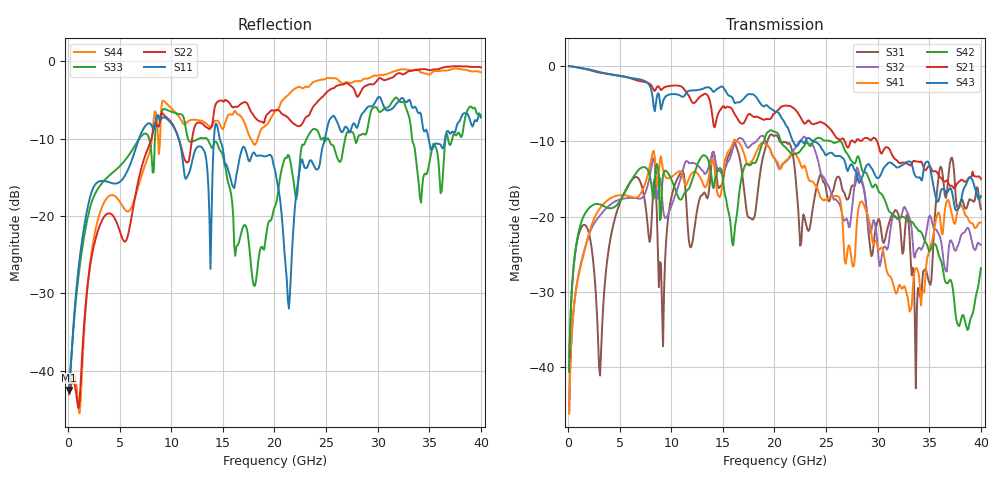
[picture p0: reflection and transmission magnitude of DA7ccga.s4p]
! ADC12DJ3200QML-SP
! 196-pin NWE package
! CCGA Ceramic Package with columns (ceramic column grid array)
! Texas Instruments 4/21/2021
! Single-ended  S-parameters
! PORT#  PORT_NAME  NET_NAME
! PORT1:  DAxN.DIEBUMP DAxN
! PORT2:  DAxN.BGA  DAxN
! PORT3:  DAxP.DIEBUMP DAxP
! PORT4:  DAxP.BGA  DAxP
! Touchstone Ver. 1.0
! Number of ports is 4
# Hz	S	MA	R	50.000000
! SCATTERING PARAMETERS  :
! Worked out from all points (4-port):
!   400 points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, 100 MHz to 40 GHz, reference 50 ohm
!   strongest paths, dB at 100 MHz, 10.1 GHz, 20.1 GHz, 30.1 GHz, 40 GHz:
!     S43: -0.1, -3.8, -6.1, -14.8, -17.3
!     S21: -0.1, -2.6, -6.2, -10.7, -15.0
!     S42: -40.6, -15.4, -8.8, -16.7, -26.8
!     S41: -46.1, -14.7, -12.5, -24.4, -20.8
!     S32: -46.1, -18.3, -12.5, -25.8, -23.8
!     S31: -40.5, -16.9, -9.2, -20.3, -19.0
!   lowest |S11| = -42.5 dB at 100 MHz (marker M1), VSWR 1.02, Z = 50.7 + j0.122 ohm
!   |S11| at or under -10 dB: start of sweep to 6.865 GHz; 10.72 GHz to 14.14 GHz (3.417 GHz wide, 27.5 % of centre); 14.7 GHz to 24.88 GHz (10.18 GHz wide, 51.5 % of centre)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
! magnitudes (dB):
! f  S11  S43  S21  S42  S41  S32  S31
! 100 MHz  -42.5  -0.1  -0.1  -40.6  -46.1  -46.1  -40.5
! 8.3 GHz  -8.8  -5.5  -3.2  -17.6  -11.3  -12.2  -15.5
! 9.2 GHz  -7.2  -4.8  -3.0  -14.5  -13.8  -19.0  -37.2
! 21.4 GHz  -32.0  -8.6  -5.3  -11.3  -12.2  -12.3  -10.2
! 32.9 GHz  -5.2  -12.7  -13.0  -20.6  -30.6  -19.5  -19.7
! 33.7 GHz  -6.0  -14.7  -12.7  -21.4  -26.8  -24.8  -42.8
! 40 GHz  -7.1  -17.3  -15.0  -26.8  -20.8  -23.8  -19.0
